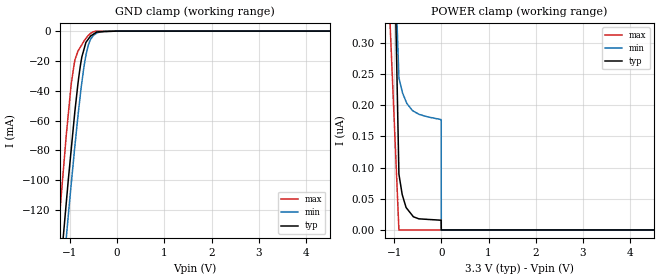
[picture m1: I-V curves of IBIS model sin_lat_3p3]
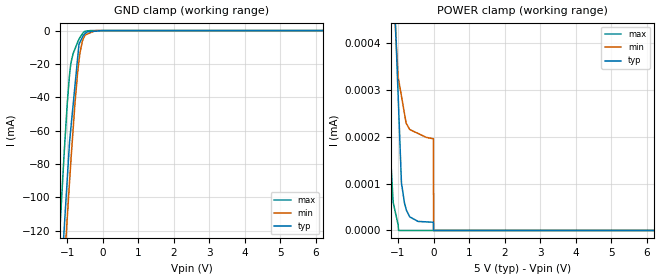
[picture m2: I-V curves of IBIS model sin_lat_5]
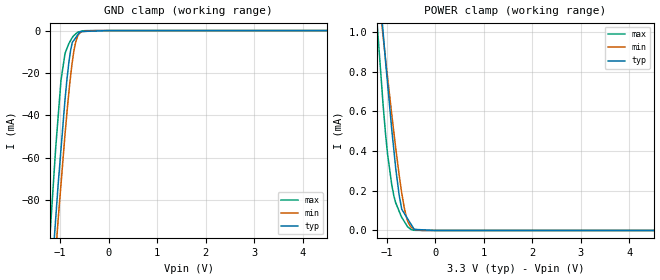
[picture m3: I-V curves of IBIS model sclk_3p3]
|Texas Instruments Incorporated
| 16-channel, 16-Bit ES-PWM LED driver with full self diagnosis for LED
| 7bit Dot Correction and 7bit Global Brightness Control
| Marketing part#   Digital Voltage Range   Package-type   #pins
| TLC5948DBQR   3.0V-5.5V   SO   24
| TLC5948DBQ   3.0V-5.5V   SO   24
| TLC5948PWPR   3.0V-5.5V   HTSSOP   24
| TLC5948PWP   3.0V-5.5V   HTSSOP   24
[IBIS Ver]   3.2
[File name]   tlc5948.ibs
|SIMDE Ver   V3.0 - 201101 - RHL4 - Build 457
[File Rev]   1.0
[Date]   8/19/2011
[Source]
| Texas Instruments Incorporated.
| Analog-eLab Design Center, HPA
| 12500 TI Blvd
| Dallas, TX -75243
| e-mail: elab_scm_ibis@list.ti.com
[Notes]   Revision History:
| Rev 1.0: 8/19/2011
| - Initial version of the model
| - Model generated from simulations in TISPICE
| - Model matched to SPICE simulation
| - C_comp although listed in numerical order of value are
|   obtained from varying PVT conditions. For PVT conditions for
|   each specific value refer the buffer description under
|   respective [Model]. IBIS model user is responsible for using
|   appropriate C_comp to simulate for Signal Integrity.
| - Model names with a trailing _3p3 contains the model for
|   3.3V [3.0V and 3.6V]. Model names with a trailing _5 contains
|   the model for 5.0V [4.5V and 5.5V].
[Disclaimer]
| This model is designed as an aid for customers of Texas Instruments.
| TI and its licensors and suppliers make no warranties, either expressed
| or implied, with respect to this  model, including the warranties of
| merchantability or fitness for a particular purpose. The model is
| provided solely on an "as is" basis. The entire risk as to its quality
| and performance is with the customer.
[Copyright]
 (C) Copyright 2011 Texas Instruments Incorporated.All rights reserved.
|   TLC5948DBQ
[Component]   TLC5948DBQ
[Manufacturer]   TI
[Package]   |24 SO   -  DBQ package
|   typ   min   max
R_pkg   0.10379   0.06407   0.13791
L_pkg   3.00792nH   2.01896nH   4.31720nH
C_pkg   0.44465pF   0.36333pF   0.58019pF
[Pin]  signal_name   model_name   R_pin   L_pin   C_pin
1   GND   GND   0.03884   4.62562nH  0.76447pF
2   SIN   SIN_LAT   0.11743   3.67071nH  0.55150pF
3   SCLK   SCLK   0.10484   2.84963nH  0.41463pF
4   LAT   SIN_LAT   0.07621   2.24154nH  0.37416pF
5   OUT0   TERM   0.10005   2.69207nH  0.39626pF
6   OUT1   TERM   0.09408   2.57858nH  0.39245pF
7   OUT2   TERM   0.09625   2.62158nH  0.39568pF
8   OUT3   TERM   0.10597   2.81035nH  0.40582pF
9   OUT4   TERM   0.12173   3.11974nH  0.42371pF
10   OUT5   TERM   0.13791   3.50503nH  0.44866pF
11   OUT6   TERM   0.13676   4.06238nH  0.57388pF
12   OUT7   TERM   0.12300   4.31720nH  0.57944pF
13   OUT8   TERM   0.12177   4.29308nH  0.58019pF
14   OUT9   TERM   0.12928   3.91484nH  0.56923pF
15   OUT10   TERM   0.12141   3.18058nH  0.43620pF
16   OUT11   TERM   0.10103   2.71823nH  0.40641pF
17   OUT12   TERM   0.08156   2.34561nH  0.38274pF
18   OUT13   TERM   0.06750   2.08343nH  0.36749pF
19   OUT14   TERM   0.06407   2.01896nH  0.36333pF
20   OUT15   TERM   0.07321   2.18471nH  0.37080pF
21   GSCLK   GSCLK   0.09141   2.52719nH  0.39096pF
22   SOUT   SOUT   0.10010   2.75826nH  0.40832pF
23   IREF   TERM   0.11772   3.68057nH  0.55049pF
24   VCC   POWER   0.11616   4.17845nH  0.56582pF
|   TLC5948PWP
[Component]   TLC5948PWP
[Manufacturer]   TI
[Package]   |24 HTSSOP -  PWP package
|   typ   min   max
R_pkg   0.25119   0.19031   0.33850
L_pkg   1.97898nH   1.46611nH   2.82829nH
C_pkg   0.30064pF   0.23684pF   0.40102pF
[Pin]  signal_name   model_name   R_pin   L_pin   C_pin
1   GND   GND   0.09525   1.86637nH  0.57461pF
2   SIN   SIN_LAT   0.24307   1.92508nH  0.31584pF
3   SCLK   SCLK   0.24536   1.89969nH  0.25893pF
4   LAT   SIN_LAT   0.20650   1.57899nH  0.25792pF
5   OUT0   TERM   0.26680   2.07602nH  0.25783pF
6   OUT1   TERM   0.25538   1.98244nH  0.25531pF
7   OUT2   TERM   0.25977   2.01874nH  0.27946pF
8   OUT3   TERM   0.27899   2.18118nH  0.26881pF
9   OUT4   TERM   0.31687   2.54037nH  0.34071pF
10   OUT5   TERM   0.33850   2.82829nH  0.40102pF
11   OUT6   TERM   0.30474   2.54792nH  0.38836pF
12   OUT7   TERM   0.25740   2.04818nH  0.31590pF
13   OUT8   TERM   0.23235   1.79747nH  0.25054pF
14   OUT9   TERM   0.25635   1.99243nH  0.28219pF
15   OUT10   TERM   0.28040   2.19205nH  0.27227pF
16   OUT11   TERM   0.25987   2.02191nH  0.26186pF
17   OUT12   TERM   0.21884   1.68280nH  0.26411pF
18   OUT13   TERM   0.19204   1.46611nH  0.23684pF
19   OUT14   TERM   0.19031   1.49620nH  0.29109pF
20   OUT15   TERM   0.21671   1.81898nH  0.34937pF
21   GSCLK   GSCLK   0.23833   1.83935nH  0.35599pF
22   SOUT   SOUT   0.23049   1.77446nH  0.35276pF
23   IREF   TERM   0.23718   1.82886nH  0.35692pF
24   VCC   POWER   0.22661   1.74219nH  0.35082pF
|   Model Selectors
[Model Selector] SIN_LAT
sin_lat_3p3   3.3V digital input
sin_lat_5   5.0V digital input
[Model Selector] SCLK
sclk_3p3   3.3V digital input
sclk_5   5.0V digital input
[Model Selector] GSCLK
gsclk_3p3   3.3V digital input
gsclk_5   5.0V digital input
[Model Selector] SOUT
sout_3p3   3.3V digital output
sout_5   5.0V digital output
[Model Selector] TERM
term_3-3V   3.3V nominal termination
term_5-0V   5.0V nominal termination
[Model] term_3-3V
Model_type Terminator
C_comp   1.0e-20F  1.0e-20F  1.0e-20F
|   typ   min   max
[Voltage Range]   3.3V   3.0V   3.6V
[POWER Clamp Reference]   3.3V   3.0V   3.6V
[GND Clamp Reference]   0V   0V   0V
|Ambient Temperature   25   85   -40
|Junction Temperature
[Temperature Range]   90   150   -40
[Model] term_5-0V
Model_type Terminator
C_comp   1.0e-20F  1.0e-20F  1.0e-20F
|   typ   min   max
[Voltage Range]   5.0V   4.5V   5.5V
[POWER Clamp Reference]   5.0V   4.5V   5.5V
[GND Clamp Reference]   0V   0V   0V
|Ambient Temperature   25   85   -40
|Junction Temperature
[Temperature Range]   90   150   -40
| Models and submodels in the file (10): sin_lat_3p3 (Input), sin_lat_5 (Input), sclk_3p3 (Input), sclk_5 (Input), gsclk_3p3 (Input), gsclk_5 (Input), sout_3p3 (Output), sout_5 (Output), term_3-3V (Terminator), term_5-0V (Terminator)
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|   sin_lat_3p3 Model
[Model]   sin_lat_3p3
Model_type   Input
Vinl = 0.99
Vinh = 2.31
|   typ   min   max
|   (nom PVT)   (fast PVT)   (slow PVT)
|C_comp from frequency sweep method (F=16.5MHz)
|Average
|C_comp   3.080e-12   2.839e-12   3.394e-12
|C_comp from LC tank measurement(L=1nH)
|Average
|Resonant Frequency(Hz)   4.080e+09   4.110e+09   3.870e+09
C_comp   1.523e-12   1.501e-12   1.693e-12
| Where nom  PVT is Nominal Process, 3.3V, 90C
|   Fast PVT is Strong Process,  3.6V, -40C
|   Slow PVT is Weak Process,   3V, 150C
[Model Spec]
|Subparameter   typ   min   max
Vinl   0.99   0.9   1.08
Vinh   2.31   2.1   2.52
[Voltage Range]   3.3   3   3.6
|Ambient Temperature   25   85   -40
|Junction Temperature
[Temperature Range]   90   150   -40
[Power Clamp Reference]   3.3   3   3.6
[GND Clamp Reference]   0   0   0
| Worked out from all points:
|   GND clamp passes 1 mA (typ) near -0.45 V on its own axis
[GND Clamp]
|   Voltage   I(typ)   I(min)   I(max)
-3.3V     -997.8mA   -999.1mA   -1.011A
-1.256V   -180.5mA   -203.3mA   -138.4mA
-1.215V   -164.9mA   -187.9mA   -122.6mA
-1.076V   -115.1mA   -138.5mA   -69.74mA
-1.038V   -101.3mA   -125.1mA   -57.13mA
-972mV    -79.44mA   -102.6mA   -35.46mA
-896.4mV  -54.51mA   -77.77mA   -19.59mA
-778.8mV  -23.39mA   -42.79mA   -10.82mA
-654mV    -7.274mA   -15.29mA   -4.645mA
-504mV    -2.122mA   -2.933mA   -467.5uA
-171mV    -240.9uA   -9.56uA    -8.997uA
6.6V      0A         0A         0A
[POWER Clamp]
|   Voltage   I(typ)   I(min)   I(max)
-3.3V     56.68uA    44.55uA    72.09uA
-1.294V   1.588uA    1.104uA    699.7nA
-897.6mV  89.57nA    245.4nA    0A
-897mV    89.28nA    244nA      0A
-828.3mV  56.85nA    222nA      0A
-745.8mV  36.02nA    205.8nA    0A
-732mV    34.69nA    203.2nA    0A
-590.7mV  21.13nA    190.5nA    0A
-468mV    17.8nA     185.4nA    0A
-3mV      15.62nA    177.1nA    0A
0V        0A         0A         0A
6.6V      0A         0A         0A
|   sin_lat_5 Model
[Model]   sin_lat_5
Model_type   Input
Vinl = 1.5
Vinh = 3.5
|   typ   min   max
|   (nom PVT)   (fast PVT)   (slow PVT)
|C_comp from frequency sweep method (F=16.5MHz)
|Average
|C_comp   2.983e-12   2.727e-12   3.268e-12
|C_comp from LC tank measurement(L=1nH)
|Average
|Resonant Frequency(Hz)   4.140e+09   4.190e+09   3.890e+09
C_comp   1.479e-12   1.444e-12   1.676e-12
| Where nom  PVT is Nominal Process, 5V, 90C
|   Fast PVT is Strong Process,  5.5V, -40C
|   Slow PVT is Weak Process,   4.5V, 150C
[Model Spec]
|Subparameter   typ   min   max
Vinl   1.5   1.35   1.65
Vinh   3.5   3.15   3.85
[Voltage Range]   5   4.5   5.5
|Ambient Temperature   25   85   -40
|Junction Temperature
[Temperature Range]   90   150   -40
[Power Clamp Reference]   5   4.5   5.5
[GND Clamp Reference]   0   0   0
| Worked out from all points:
|   GND clamp passes 1 mA (typ) near -0.45 V on its own axis
[GND Clamp]
|   Voltage   I(typ)   I(min)   I(max)
-5V       -1.705A    -1.689A    -1.759A
-1.216V   -165.5mA   -188.2mA   -122.3mA
-1.089V   -119.9mA   -142.9mA   -74.3mA
-1.017V   -94.98mA   -117.9mA   -49.54mA
-935mV    -66.64mA   -90.34mA   -26.33mA
-891mV    -56.94mA   -76.04mA   -18.88mA
-778.5mV  -32.15mA   -42.47mA   -10.78mA
-670mV    -8.245mA   -17.92mA   -5.263mA
-576mV    -4.122mA   -6.514mA   -2.044mA
-495mV    -1.687mA   -2.656mA   -372.8uA
-193.5mV  -329.1uA   -15.9uA    -2.481uA
10V       0A         0A         0A
[POWER Clamp]
|   Voltage   I(typ)   I(min)   I(max)
-5V       90.18uA    70.35uA    115.2uA
-1.315V   1.97uA     1.181uA    473.3nA
-1.232V   1.13uA     786.3nA    187.8nA
-1.139V   571.9nA    521.4nA    60.2nA
-999mV    291.2nA    328.9nA    12.44nA
-984.5mV  262.1nA    322.6nA    0A
-905mV    102.1nA    287.6nA    0A
-765mV    43.32nA    228.4nA    0A
-435mV    19.31nA    207.4nA    0A
-4.5mV    17.6nA     196.2nA    0A
0V        0A         0A         0A
10V       0A         0A         0A
|   sclk_3p3 Model
[Model]   sclk_3p3
Model_type   Input
Vinl = 0.99
Vinh = 2.31
|   typ   min   max
|   (nom PVT)   (fast PVT)   (slow PVT)
|C_comp from frequency sweep method (F=33MHz)
|Average
|C_comp   8.200e-13   7.978e-13   8.823e-13
|C_comp from LC tank measurement(L=1nH)
|Average
|Resonant Frequency(Hz)   6.720e+09   6.850e+09   6.560e+09
C_comp   5.615e-13   5.404e-13   5.892e-13
| Where nom  PVT is Nominal Process, 3.3V, 90C
|   Fast PVT is Strong Process,  3.6V, -40C
|   Slow PVT is Weak Process,   3V, 150C
[Model Spec]
|Subparameter   typ   min   max
Vinl   0.99   0.9   1.08
Vinh   2.31   2.1   2.52
[Voltage Range]   3.3   3   3.6
|Ambient Temperature   25   85   -40
|Junction Temperature
[Temperature Range]   90   150   -40
[Power Clamp Reference]   3.3   3   3.6
[GND Clamp Reference]   0   0   0
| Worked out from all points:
|   GND clamp passes 1 mA (typ) near -0.60 V on its own axis
|   POWER clamp passes 1 mA (typ) near -1.08 V on its own axis
[GND Clamp]
|   Voltage   I(typ)   I(min)   I(max)
-3.3V     -902.9mA   -878.4mA   -959mA
-1.218V   -130.3mA   -145.1mA   -100.9mA
-1.087V   -88.41mA   -104.6mA   -55.07mA
-1.04V    -73.15mA   -89.79mA   -41.12mA
-979.2mV  -56.04mA   -72.58mA   -23.48mA
-896.4mV  -32.6mA    -49.01mA   -10.8mA
-815.1mV  -14.68mA   -28.87mA   -6.071mA
-745.8mV  -5.578mA   -14.79mA   -3.285mA
-720mV    -4.761mA   -10.57mA   -2.463mA
-637.2mV  -2.136mA   -2.776mA   -782.3uA
-285mV    -221.9uA   -4.709uA   -7.129uA
6.6V      0A         0A         0A
[POWER Clamp]
|   Voltage   I(typ)   I(min)   I(max)
-3.3V     7.852mA    6.423mA    9.069mA
-1.213V   1.39mA     1.29mA     1.087mA
-1.171V   1.267mA    1.194mA    947.7uA
-1.076V   995.2uA    976.9uA    630.4uA
-986.4mV  743.2uA    775.1uA    386.6uA
-896.4mV  502.3uA    578.5uA    226uA
-745.8mV  176.7uA    278.4uA    96.06uA
-693mV    106.9uA    188.3uA    66.25uA
-636mV    84.37uA    108.4uA    43.52uA
-504mV    32.11uA    17.53uA    5.325uA
-3.3mV    0A         18.73nA    0A
6.6V      0A         0A         0A
